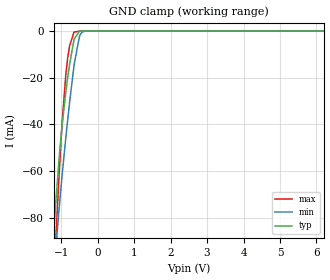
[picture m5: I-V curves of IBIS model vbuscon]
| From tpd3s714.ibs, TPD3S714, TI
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|   vbuscon Model
[Model]   vbuscon
Model_type   Terminator
|   typ   min   max
|   (nom PVT)   (fast PVT)   (slow PVT)
C_comp   3.240e-10   3.192e-10   3.418e-10
| Where nom  PVT is Nominal Process, 5V, 40C
|   Fast PVT is Strong Process,  5.5V, -40C
|   Slow PVT is Weak Process,   4.5V, 125C
[Voltage Range]   5   4.5   5.5
|Junction Temperature
[Temperature Range]   40   125   -40
[Power Clamp Reference]   5   4.5   5.5
[GND Clamp Reference]   0   0   0
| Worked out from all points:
|   GND clamp passes 1 mA (typ) near -0.54 V on its own axis
[GND Clamp]
|   Voltage   I(typ)   I(min)   I(max)
-5V       -1.517A    -1.407A    -1.76A
-1.24V    -95.51mA   -113.6mA   -120mA
-1.15V    -74.29mA   -94.4mA    -90.54mA
-1.058V   -55.23mA   -76.72mA   -62.47mA
-965mV    -39.23mA   -60.63mA   -37.69mA
-869.5mV  -25.96mA   -45.52mA   -18.43mA
-820mV    -20mA      -38.12mA   -11.48mA
-770.5mV  -14.53mA   -31.01mA   -6.498mA
-639.5mV  -3.367mA   -14.03mA   -432.3uA
-500mV    -128.3uA   -2.482mA   -9.375uA
-329mV    -1.124uA   -57.38uA   -106.9nA
10V       0A         0A         0A
[POWER Clamp]
|   Voltage   I(typ)   I(min)   I(max)
-5V       0A         0A         0A
0V        0A         0A         0A
10V       0A         0A         0A
